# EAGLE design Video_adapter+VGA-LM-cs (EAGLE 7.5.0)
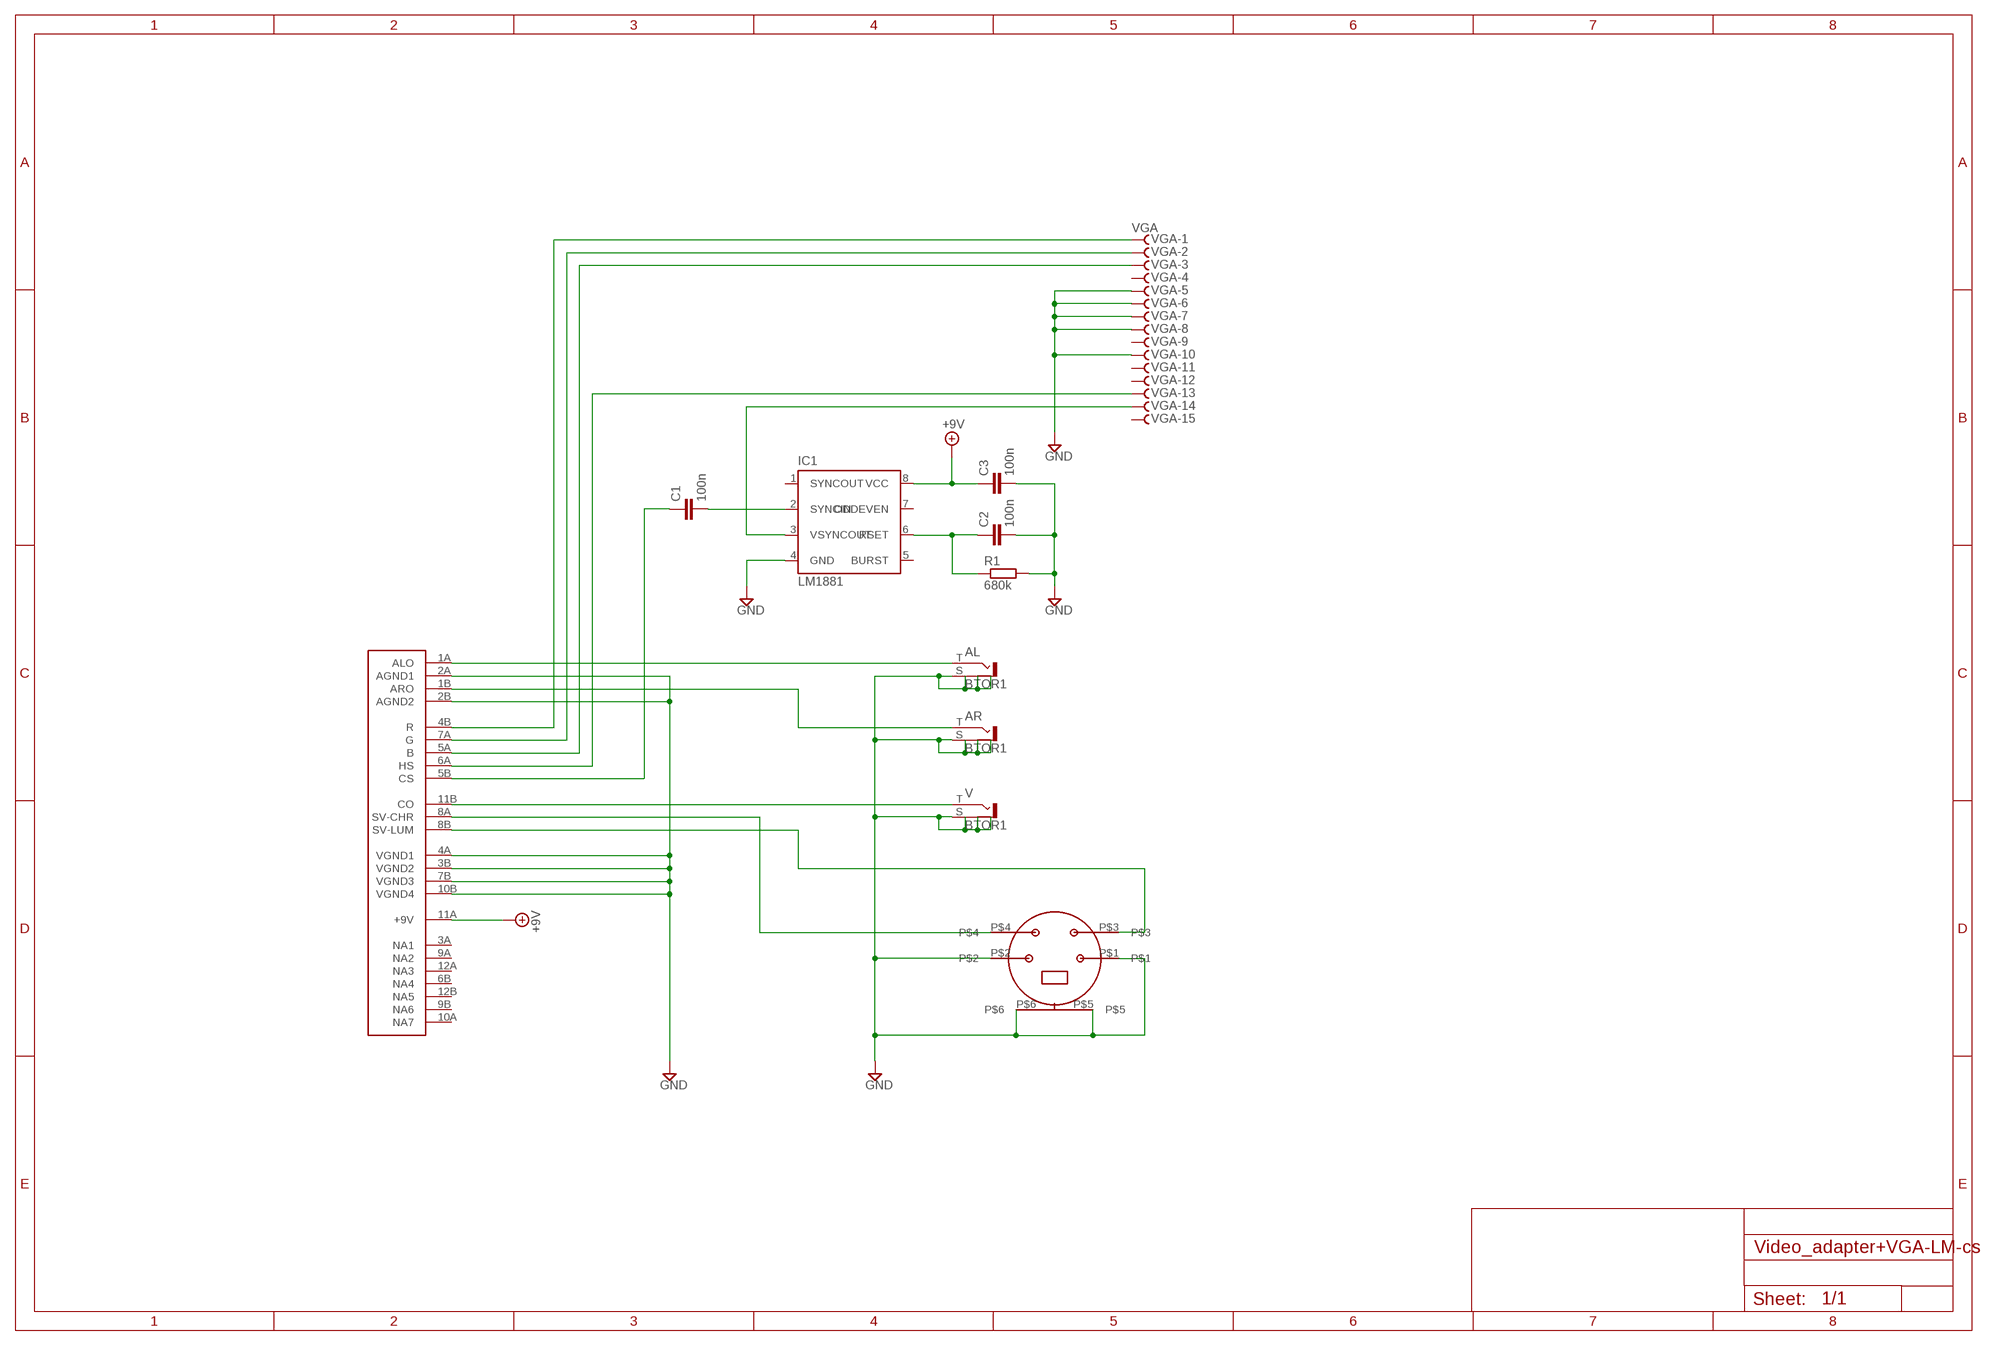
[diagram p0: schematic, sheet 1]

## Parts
AL  BTOR1  [BTOR1]
AR  BTOR1  [BTOR1]
C1  100n  C-EUC0805  [C0805]
C2  100n  C-EUC0805  [C0805]
C3  100n  C-EUC0805  [C0805]
CONN1  24POSCECARDEDGE  [24POSEDGECARD]
IC1  LM1881  LM1881SOIC8  [SOIC8]
R1  680k  R-EU_R0805  [R0805]
U$1  MINI_DIN_4V  [M_DIN4_V1]
V  BTOR1  [BTOR1]
VGA  VGA  HF15VS  [HDF15V]

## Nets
+9V: C3.1 CONN1.11A(+9V) IC1.8(VCC)
AUDIO-LEFT: AL.T CONN1.1A(ALO)
AUDIO-RIGHT: AR.T CONN1.1B(ARO)
B: CONN1.5A(B) VGA.3
COMPOSIT: CONN1.11B(CO) V.T
CSYNC: C1.1 CONN1.5B(CS)
G: CONN1.7A(G) VGA.2
GND: AL.S AL.S@1 AL.S@2 AL.S@3 AR.S AR.S@1 AR.S@2 AR.S@3 C2.2 C3.2 CONN1.2A(AGND1) CONN1.2B(AGND2) CONN1.3B(VGND2) CONN1.4A(VGND1) CONN1.7B(VGND3) CONN1.10B(VGND4) IC1.4(GND) R1.2 U$1.P$1 U$1.P$2 U$1.P$5 U$1.P$6 V.S V.S@1 V.S@2 V.S@3 VGA.5 VGA.6 VGA.7 VGA.8 VGA.10
HSYNC: CONN1.6A(HS) VGA.13
N$13: C1.2 IC1.2(SYNCIN)
N$19: C2.1 IC1.6(RSET) R1.1
R: CONN1.4B(R) VGA.1
SV-CHROMA: CONN1.8A(SV-CHR) U$1.P$4
SV-LUMA: CONN1.8B(SV-LUM) U$1.P$3
VSYNC: IC1.3(VSYNCOUT) VGA.14
Unconnected: CONN1.3A(NA1) CONN1.6B(NA4) CONN1.9A(NA2) CONN1.9B(NA6) CONN1.10A(NA7) CONN1.12A(NA3) IC1.1(SYNCOUT) IC1.5(BURST) IC1.7(ODDEVEN) VGA.4 VGA.9 VGA.11 VGA.12 VGA.15

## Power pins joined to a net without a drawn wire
NA5: CONN1.12B(NA5)

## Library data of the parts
AL AR V = con-lumberg:BTOR1: RCA connectors according to JEITA RC-5231 Cinch RCA-Einbaukupplung nach JEITA RC-5231, stehende Ausführung Source: http://www.lumberg.de/Produkte/PDFs/BTOR1.pdf; MPN: BTOR 1; OC_FARNELL: 1217030; OC_NEWARK: 96K7172
C1-C3 = rcl:C-EU: CAPACITOR, European symbol
CONN1 = jaguar:24POSCE
IC1 = lm1881:LM1881
R1 = rcl:R-EU_: RESISTOR, European symbol
U$1 = mini_din:MINI_DIN_4V
VGA = con-subd:HF15?S: SUB-D; OC_FARNELL: unknown; OC_NEWARK: unknown

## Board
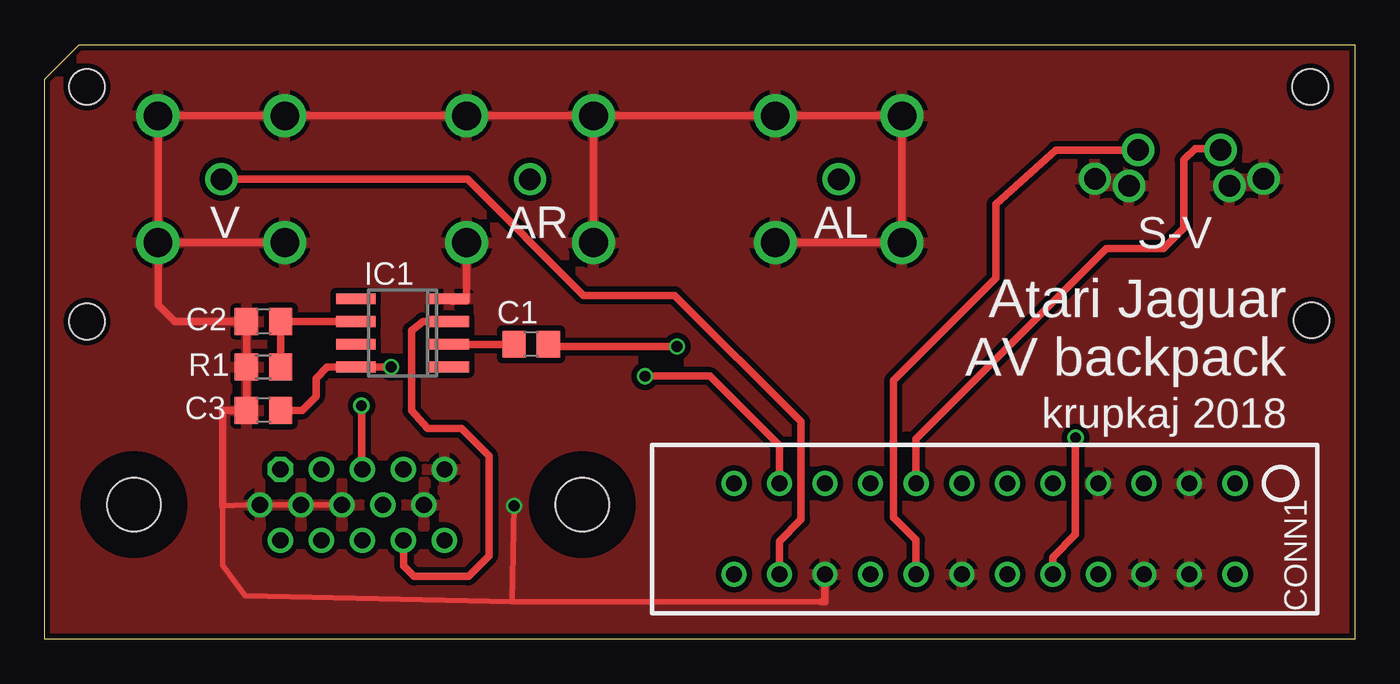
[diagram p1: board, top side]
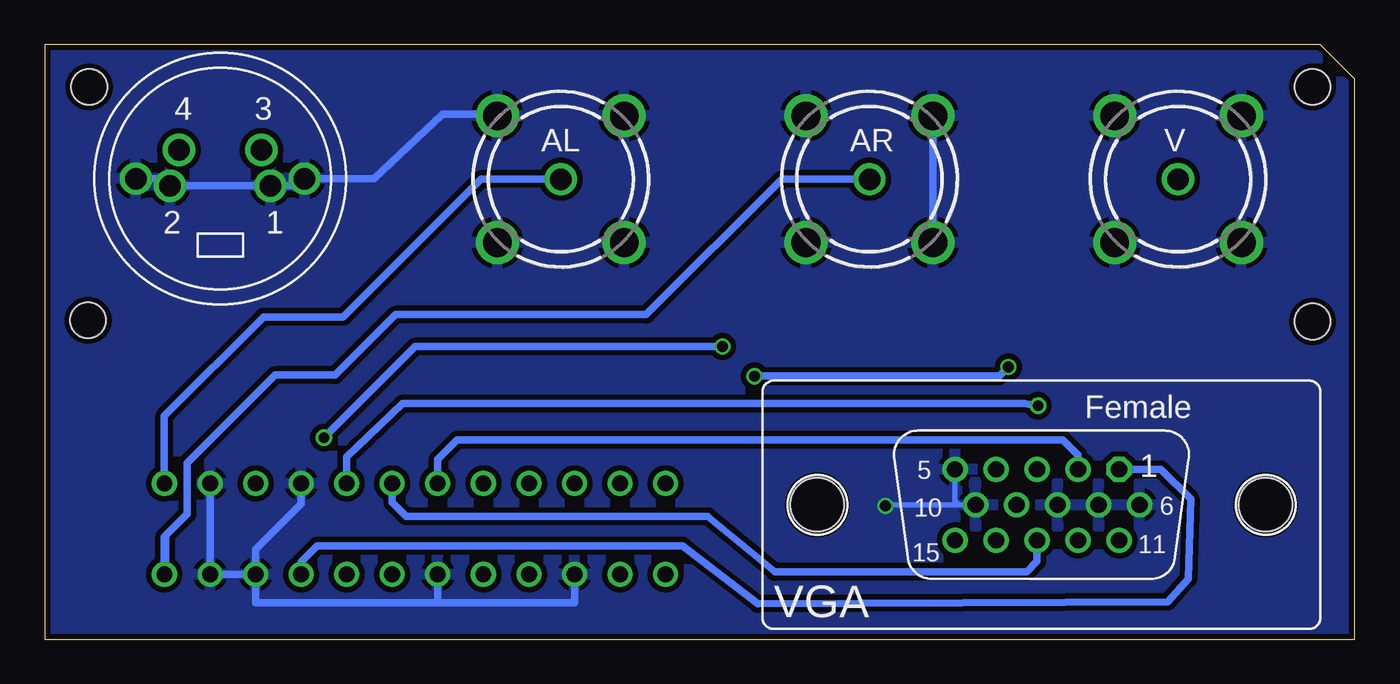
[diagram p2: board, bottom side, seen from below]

Size 73.02 x 33.15 mm. Coordinates in mm from the lower left corner, seen from the top.
Outline: 1.9,33.15 73.02,33.15 73.02,0 0,0 0,31.24 1.9,33.15
Copper layers (1*16): Top 0.035mm / dielectric 1.5mm / Bottom 0.035mm
Design rules "SeeedStudio_2layer_DRU_no_angle_20140221": minimum track width 6mil, minimum drill 12mil, track to track 6mil, track to pad 6mil, pad to pad 6mil, via to via 6mil, smd to smd 0mil, copper to edge 10mil, drill to drill 10mil, minimum pad ring 10mil, minimum via ring 6mil, stop-mask expansion 2mil, vias tented up to drill 100mil, thermal gap 10mil
Holes 2 mm at 2.35,30.8 70.55,30.8 70.61,17.78 2.35,17.72

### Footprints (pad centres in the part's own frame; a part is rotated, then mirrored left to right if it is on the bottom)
BTOR1 = drill 1.6 pad 2.2: S -5,0; S@1 0,5; S@2 5,0; S@3 0,-5 | drill 1.2 pad 1.6: T 0,0
C0805 = smd 1.3 x 1.5: 1 -0.95,0; 2 0.95,0
24POSEDGECARD = drill 0.889: 1A -13.97,-0.94; 1B -13.97,4.14; 2A -11.43,-0.94; 2B -11.43,4.14; 3A -8.89,-0.94; 3B -8.89,4.14; 4A -6.35,-0.94; 4B -6.35,4.14; 5A -3.81,-0.94; 5B -3.81,4.14; 6A -1.27,-0.94; 6B -1.27,4.14; 7A 1.27,-0.94; 7B 1.27,4.14; 8A 3.81,-0.94; 8B 3.81,4.14; 9A 6.35,-0.94; 9B 6.35,4.14; 10A 8.89,-0.94; 10B 8.89,4.14; 11A 11.43,-0.94; 11B 11.43,4.14; 12A 13.97,-0.94; 12B 13.97,4.14
SOIC8 = smd 0.6 x 2.2: 1 -3.175,-3.87; 2 -1.905,-3.87; 3 -0.635,-3.87; 4 0.635,-3.87; 5 0.635,1.33; 6 -0.635,1.33; 7 -1.905,1.33; 8 -3.175,1.33
R0805 = smd 1.3 x 1.5: 1 -0.95,0; 2 0.95,0
M_DIN4_V1 = drill 1.2 pad 1.676: P$1 2.8,-0.5; P$2 -2.8,-0.5; P$3 2.3,1.5; P$4 -2.3,1.5 | drill 1.2 pad 1.422: P$5 -4.7,-0.1; P$6 4.7,-0.1
HDF15V = drill 0.9 octagon: 1 4.329,1.98 | drill 0.9: 2 2.043,1.98; 3 -0.243,1.98; 4 -2.529,1.98; 5 -4.815,1.98; 6 5.472,0; 7 3.186,0; 8 0.9,0; 9 -1.386,0; 10 -3.672,0; 11 4.329,-1.98; 12 2.043,-1.98; 13 -0.243,-1.98; 14 -2.529,-1.98; 15 -4.815,-1.98 | hole 3: -12.5,0; 12.5,0

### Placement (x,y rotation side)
AL  44.26,25.65 45 bottom
AR  27.05,25.65 45 bottom
C1  27.11,16.45 180 top
C2  12.19,17.72 180 top
C3  12.19,12.76 180 top
CONN1  52.39,7.75 180 top
IC1  18.67,18.35 90 top
R1  12.19,15.18 180 top
U$1  63.25,25.78 0 bottom
V  9.84,25.65 45 bottom
VGA  17.46,7.49 0 bottom

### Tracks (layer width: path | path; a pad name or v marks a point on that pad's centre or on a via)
+9V  (via drill 0.6)
  Top 0.406: v33.46,14.67 37.08,14.67 40.96,10.79 CONN1.11A | v19.3,15.18 IC1.8 15.75,15.18 15.11,14.54 15.11,13.53 14.35,12.76 C3.1
  Bottom 0.406: v33.46,14.67 19.81,14.67 v19.3,15.18
AUDIO-LEFT
  Bottom 0.406: AL.T 48.7,25.65 56.39,17.97 60.83,17.97 66.36,12.45 CONN1.1A
AUDIO-RIGHT
  Bottom 0.406: AR.T 31.94,25.65 39.5,18.1 53.47,18.1 56.83,14.73 60.2,14.73 65.09,9.84 65.09,6.99 66.29,5.78 | 66.29,5.78 66.29,3.67 | CONN1.1B 66.36,5.71 66.29,5.78
B  (via drill 0.6)
  Top 0.406: v17.65,13.02 17.65,9.53 VGA.3
  Bottom 0.406: v17.65,13.02 18.41,13.14 53.09,13.14 55.63,10.73 56.2,10.16 CONN1.5A
COMPOSIT
  Top 0.406: V.T 23.56,25.65 30.04,19.18 35.12,19.18 42.16,12.13 42.16,6.67 40.96,5.46 CONN1.11B
CSYNC  (via drill 0.6)
  Top 0.406: 27.75,16.45 C1.1 27.87,16.32 v35.24,16.32 | v57.47,11.24 57.47,5.84 56.2,4.57 CONN1.5B
  Bottom 0.406: v35.24,16.32 52.39,16.32 v57.47,11.24
G
  Bottom 0.406: VGA.2 15.42,10.28 16.26,11.11 50.04,11.11 51.12,10.03 CONN1.7A
GND  (via drill 0.6)
  Top 0.305: v26.16,7.43 26.04,2.1 | 26.04,2.1 43.31,2.1 | 26.04,2.1 11.18,2.41 9.91,4.13 9.91,7.43 11.23,7.48 VGA.6 VGA.7 VGA.8
  Top 0.406: V.S@3 6.31,18.65 7.24,17.72 C2.2 R1.2 C3.2 9.91,12.76 9.91,7.43 | AR.S@3 23.52,18.88 23.5,18.86 22.67,18.86 IC1.4 | V.S@3 V.S@2 V.S@1 AR.S@2 AR.S@1 | CONN1.10B 43.5,2.1 43.31,2.1 | AR.S@1 AL.S@2 AL.S@1 AL.S AL.S@3 | AR.S@1 AR.S | V.S V.S@3
  Bottom 0.305: VGA.10 22.1,7.49 | 22.1,7.49 26.35,7.49 v26.16,7.43 | VGA.5 22.28,7.67 22.1,7.49
  Bottom 0.406: AR.S@2 AR.S@3 | CONN1.3B CONN1.2B CONN1.2A | CONN1.4A 58.74,7.56 61.28,5.02 CONN1.3B | AL.S@1 47.79,29.27 50.86,29.27 54.67,25.68 U$1.P$6 58.55,25.28 U$1.P$1 U$1.P$2 66.05,25.68 U$1.P$5 | CONN1.7B 51.12,2.03 | 51.12,2.03 61.28,2.03 CONN1.3B | CONN1.10B 43.5,2.03 51.12,2.03
  pour Top (isolate 0.305): -3.05,-3.05 77.03,-3.05 77.22,34.1 -3.17,34.42
  pour Bottom (isolate 0.305): 75.76,37.08 75.31,-1.59 -1.4,-1.71 -1.27,36.96
HSYNC
  Bottom 0.406: VGA.13 17.7,4.33 18.29,3.75 32.32,3.75 36.07,6.86 52.9,6.86 53.66,7.62 CONN1.6A
N$13
  Top 0.406: C1.2 IC1.2
N$19
  Top 0.406: IC1.6 C2.1 R1.1
R
  Bottom 0.406: VGA.1 10.81,9.47 9.14,7.81 9.27,3.37 10.41,2.1 33.27,1.97 37.46,5.21 57.85,5.21 58.74,4.32 CONN1.4B
SV-CHROMA
  Top 0.406: U$1.P$4 65.46,27.37 64.14,27.37 63.5,26.73 63.5,22.92 62.36,21.78 59.18,21.78 48.58,11.18 CONN1.8A
SV-LUMA
  Top 0.406: CONN1.8B 48.58,5.52 47.31,6.79 47.31,14.41 53.02,20.13 53.02,24.26 56.36,27.28 U$1.P$3
VSYNC
  Top 0.406: IC1.3 21.08,17.72 20.45,17.21 20.45,12.76 21.34,11.75 23.24,11.75 24.77,10.22 24.77,4.64 23.62,3.49 20.57,3.49 19.99,4.07 VGA.14

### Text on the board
tNames: V | AR | AL | S-V | Atari Jaguar / AV backpack | krupkaj 2018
